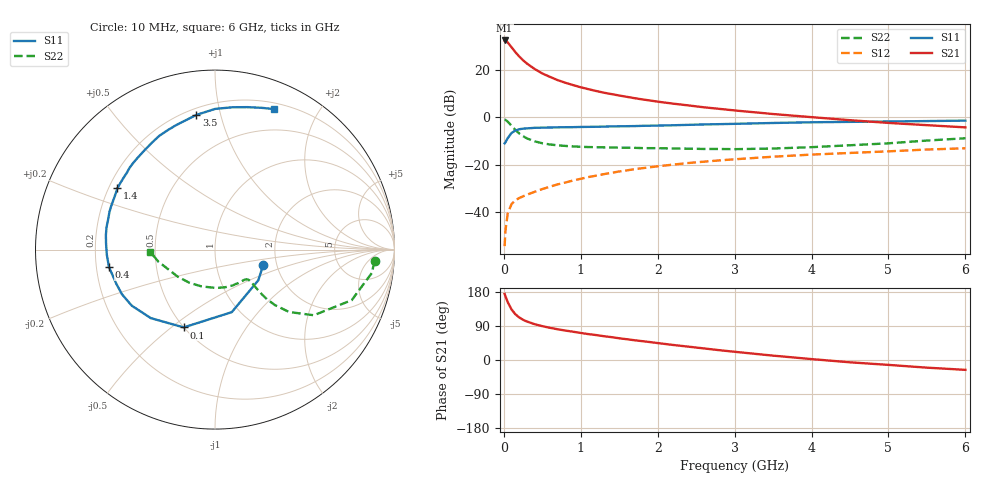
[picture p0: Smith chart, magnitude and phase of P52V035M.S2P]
! SIEMENS Small Signal Semiconductors
! BFP183
! Si NPN RF Bipolar Junction Transistor in SOT143
! VCE = 2 V  IC = 35 mA
! Common Emitter S-Parameters:  March  1996
# GHz  S  MA  R  50
!  f  S11  S21  S12  S22
! GHz  MAG  ANG  MAG  ANG  MAG  ANG  MAG  ANG
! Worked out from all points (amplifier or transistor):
!   36 points, 10 MHz to 6 GHz, reference 50 ohm
!   highest |S21| = 32.4 dB at 10 MHz (marker M1)
!   |S21| within 3 dB of that: start of sweep to 103.1 MHz
!   unconditionally stable (mu >= 1): start of sweep to 12.35 MHz; 407.5 MHz to end of sweep
!   at 250 MHz: K = 0.77, MSG = 28.7 dB, |S12| = -33.4 dB
!   at 1.4 GHz: K = 1.31, MAG = 13.3 dB, |S12| = -23.5 dB
!   at 6 GHz: K = 1.02, MAG = 3.5 dB, |S12| = -13.1 dB
!   S11 on the Smith chart (normalised r, x): 10 MHz: 1.70, -0.32; 100 MHz: 0.50, -0.55; 400 MHz: 0.25, -0.08; 1.4 GHz: 0.23, +0.27; 3.5 GHz: 0.24, +0.84; 6 GHz: 0.26, +1.47
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0.01  0.2818 -17.7  41.84 174.2  0.0019 72.6  0.8914 -4.1
0.02  0.2958 -35.3  41.45 168.9  0.0039 78.8  0.8832 -8.5
0.05  0.3608 -75.0  38.13 152.8  0.0093 69.5  0.8121 -20.3
0.1  0.4672 -111.9  30.05 133.5  0.0147 54.6  0.6609 -33.6
0.15  0.523 -133.1  23.74 120.7  0.0177 51.3  0.5397 -40.1
0.2  0.5591 -146.0  19.21 112.3  0.0197 49.1  0.4548 -42.8
0.25  0.575 -154.4  15.96 106.1  0.0214 49.8  0.3993 -43.7
0.3  0.5819 -160.9  13.62 101.6  0.0232 50.0  0.3583 -43.6
0.4  0.5988 -170.7  10.46 94.5  0.0267 52.8  0.3101 -42.9
0.5  0.6035 -177.4  8.416 89.3  0.0305 54.2  0.2824 -42.2
0.6  0.6079 176.9  7.118 84.9  0.0343 55.7  0.2663 -41.8
0.7  0.6133 172.4  6.078 81.1  0.0383 57.2  0.2555 -41.9
0.9  0.6183 164.6  4.779 74.6  0.0463 58.6  0.2426 -43.1
1.1  0.6272 157.3  3.918 68.3  0.0548 58.8  0.235 -45.5
1.4  0.6427 147.7  3.084 60.3  0.0671 58.2  0.2298 -50.5
1.7  0.6516 138.9  2.528 52.1  0.0802 56.3  0.2262 -56.9
2.2  0.6778 125.7  1.94 39.7  0.1002 52.1  0.2188 -69.4
2.8  0.7155 111.7  1.506 25.9  0.1228 46.2  0.2139 -87.4
3.5  0.7576 97.9  1.171 11.5  0.147 39.8  0.2188 -110.9
4.5  0.7993 82.9  0.868 -6.1  0.1765 30.0  0.2565 -144.0
5.5  0.8311 71.9  0.681 -20.2  0.2084 21.4  0.3224 -167.9
6  0.8492 67.2  0.612 -26.0  0.2215 16.4  0.3609 -178.0
